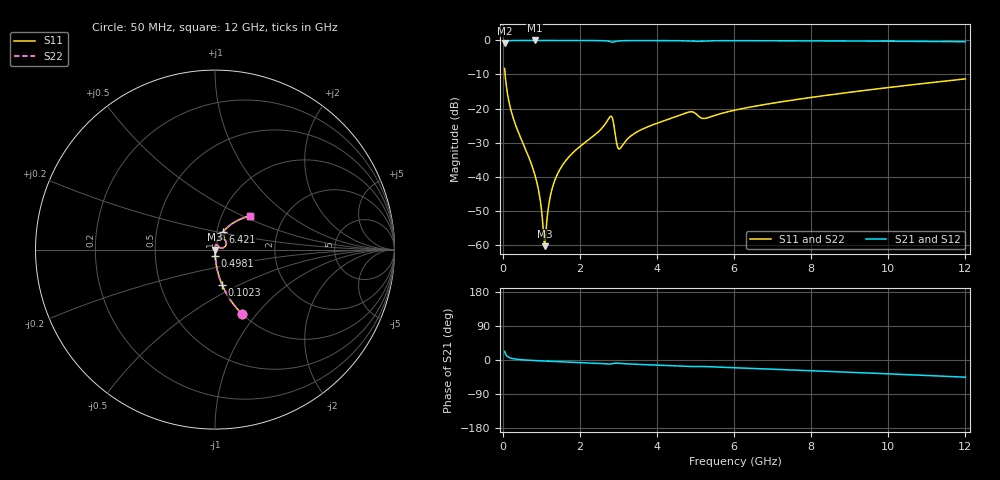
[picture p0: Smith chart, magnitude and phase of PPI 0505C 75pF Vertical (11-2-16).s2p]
# GHz S MA R 50
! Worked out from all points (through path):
!   1601 points, 50 MHz to 12 GHz, reference 50 ohm
!   highest |S21| = -0.01 dB at 834.2 MHz (marker M1); lowest = -0.7 dB at 50 MHz (marker M2)
!   group delay of S21, straight-line fit = 10.8 ps
!   lowest |S11| = -60.4 dB at 1.088 GHz (marker M3), VSWR 1.00, Z = 50.1 - j0.00775 ohm
!   |S11| at or under -10 dB: 63.3 MHz to end of sweep
!   |S22| runs from -60.4 to -8.2 dB; largest |S21 - S12| = 0
!   S11 on the Smith chart (normalised r, x): 50 MHz: 1.00, -0.84; 102.3 MHz: 1.00, -0.41; 498.1 MHz: 1.00, -0.07; 6.421 GHz: 1.07, +0.21; 12 GHz: 1.36, +0.55
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0.05  0.3889 -67.2  0.921 22.8  0.921 22.8  0.3889 -67.2
0.1022813  0.2008 -78.6  0.9793 11.3  0.9793 11.3  0.2008 -78.6
0.2441875  0.08203 -85.6  0.9961 4.1  0.9961 4.1  0.08203 -85.6
0.498125  0.03367 -88.2  0.9987 0.7  0.9987 0.7  0.03367 -88.2
0.8342188  0.01062 -87.0  0.9991 -1.5  0.9991 -1.5  0.01062 -87.0
0.94625  0.005621 -83.0  0.999 -2.1  0.999 -2.1  0.005621 -83.0
1.050812  0.001692 -59.1  0.999 -2.6  0.999 -2.6  0.001692 -59.1
1.088156  0.0009496 -4.7  0.999 -2.7  0.999 -2.7  0.0009496 -4.7
1.1255  0.001623 50.6  0.999 -2.9  0.999 -2.9  0.001623 50.6
1.245  0.005442 75.8  0.9989 -3.5  0.9989 -3.5  0.005442 75.8
1.386906  0.009856 79.7  0.9988 -4.1  0.9988 -4.1  0.009856 79.7
2.044156  0.02886 80.1  0.9979 -6.8  0.9979 -6.8  0.02886 80.1
2.783562  0.07571 51.1  0.962 -10.8  0.962 -10.8  0.07571 51.1
3.030031  0.02548 46.1  0.9849 -8.8  0.9849 -8.8  0.02548 46.1
4.038312  0.06172 73.5  0.9948 -13.7  0.9948 -13.7  0.06172 73.5
4.844938  0.08907 62.0  0.9791 -17.2  0.9791 -17.2  0.08907 62.0
5.225844  0.07136 59.5  0.9806 -17.1  0.9806 -17.1  0.07136 59.5
6.025  0.09469 67.0  0.991 -20.5  0.991 -20.5  0.09469 67.0
6.420844  0.105 66.0  0.9905 -22.1  0.9905 -22.1  0.105 66.0
8.019156  0.146 60.4  0.9856 -28.4  0.9856 -28.4  0.146 60.4
10.01331  0.2036 52.5  0.9749 -36.6  0.9749 -36.6  0.2036 52.5
12  0.2722 43.8  0.9575 -45.4  0.9575 -45.4  0.2722 43.8
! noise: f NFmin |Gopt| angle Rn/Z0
0.05  0.0003757  0.86  0.4022  0.0005747
1.372  0.003879  0.6665  3.419  0.00223
2.701  0.02001  0.8582  6.766  0.03007
4.031  0.01127  0.6641  9.836  0.006384
5.36  0.02394  0.776  13.31  0.02156
6.682  0.01529  0.6058  15.88  0.007041
8.012  0.01644  0.5713  18.6  0.006768
9.341  0.01835  0.5579  21.31  0.007209
10.67  0.02056  0.5531  23.98  0.007901
12  0.02304  0.5538  26.61  0.008788
